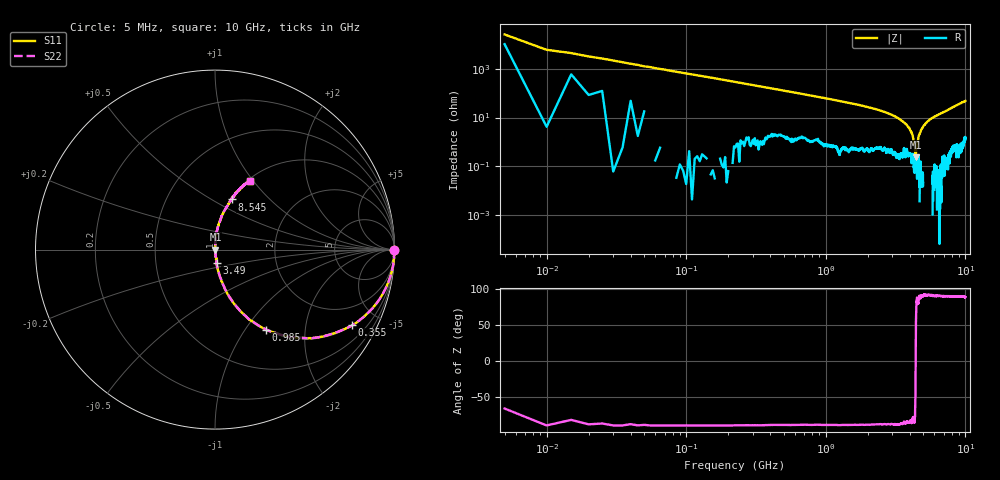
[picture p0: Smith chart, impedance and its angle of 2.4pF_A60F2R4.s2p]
! Amotech Co.,Ltd.
! http://www.amotech.co.kr/
! Part Number: A60F2R4
! These Parameters are Measured in Series Mode Connection
! Operation Temp=25[degC], DC Bias Voltage=0[V]
! Freq. Start=5[MHz] Stop=10[GHz], 2000[Steps]
! Date: Monday, July 20, 2020, 03:51:40
# GHZ S RI R 50.000000
!Freq.(Hz) S11(Real) S11(Imag) S21(Real) S21(Imag) S12(Real) S12(Imag) S22(Real) S22(Imag)
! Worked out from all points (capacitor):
!   2000 points, 5 MHz to 10 GHz, reference 50 ohm
!   read as one part in series: C = 2.47 pF near 55 MHz
!   lowest |Z| = 234 mohm at 4.405 GHz (marker M1)
!   series resonance near 4.403 GHz, so ESL is about 530 pH
!   S11 on the Smith chart (normalised r, x): 5 MHz: open; 355 MHz: 1.02, -3.61; 985 MHz: 1.01, -1.25; 3.49 GHz: 1.01, -0.15; 8.545 GHz: 1.01, +0.62; 10 GHz: 1.03, +0.96
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0.005  0.9984 -0.00358  0.00157 0.00358  0.00157 0.00358  0.9984 -0.00358
0.06  0.9913 -0.093  0.00874 0.093  0.00874 0.093  0.9913 -0.093
0.1  0.9769 -0.1503  0.0231 0.1503  0.0231 0.1503  0.9769 -0.1503
0.205  0.9096 -0.2867  0.0904 0.2867  0.0904 0.2867  0.9096 -0.2867
0.355  0.7639 -0.4217  0.2361 0.4217  0.2361 0.4217  0.7639 -0.4217
0.59  0.5355 -0.4939  0.4645 0.4939  0.4645 0.4939  0.5355 -0.4939
0.985  0.2844 -0.4454  0.7156 0.4454  0.7156 0.4454  0.2844 -0.4454
1.675  0.1077 -0.3029  0.8923 0.3029  0.8923 0.3029  0.1077 -0.3029
3.34  0.0104 -0.0883  0.9896 0.0883  0.9896 0.0883  0.0104 -0.0883
3.49  0.0087 -0.0728  0.9913 0.0728  0.9913 0.0728  0.0087 -0.0728
3.94  0.00427 -0.0384  0.9957 0.0384  0.9957 0.0384  0.00427 -0.0384
4.13  0.00222 -0.0233  0.9978 0.0233  0.9978 0.0233  0.00222 -0.0233
4.22  0.00296 -0.0143  0.997 0.0143  0.997 0.0143  0.00296 -0.0143
4.375  0.00213 -0.00334  0.9979 0.00334  0.9979 0.00334  0.00213 -0.00334
4.405  0.00232 0.000271  0.9977 -0.000271  0.9977 -0.000271  0.00232 0.000271
4.635  0.00216 0.018  0.9978 -0.018  0.9978 -0.018  0.00216 0.018
5.005  0.00146 0.0449  0.9985 -0.0449  0.9985 -0.0449  0.00146 0.0449
5.72  0.0068 0.0935  0.9932 -0.0935  0.9932 -0.0935  0.0068 0.0935
6.67  0.0227 0.1449  0.9773 -0.1449  0.9773 -0.1449  0.0227 0.1449
8.335  0.0812 0.2617  0.9188 -0.2617  0.9188 -0.2617  0.0812 0.2617
8.545  0.0925 0.2797  0.9075 -0.2797  0.9075 -0.2797  0.0925 0.2797
10  0.1958 0.381  0.8042 -0.381  0.8042 -0.381  0.1958 0.381
